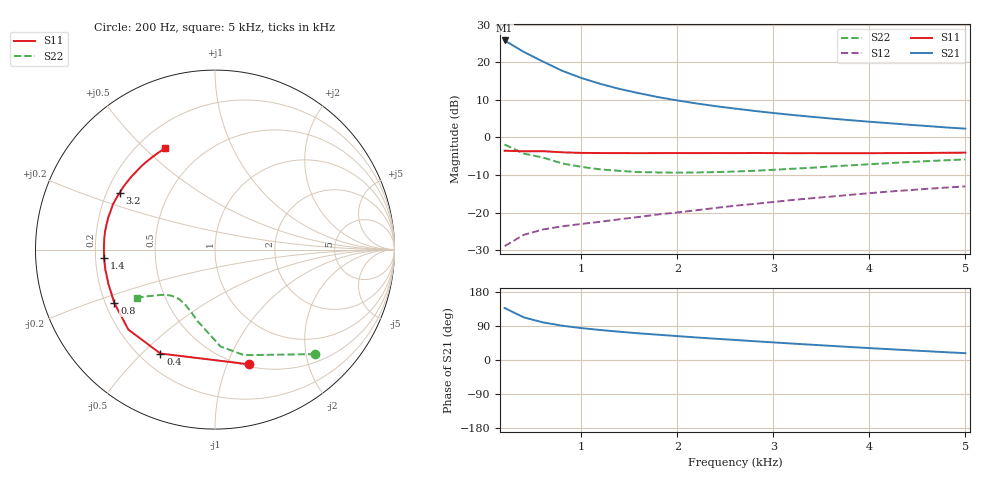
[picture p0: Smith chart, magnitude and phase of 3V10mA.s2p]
#  HZ  S  MA  R  50.0000
! Device:MCH4020
! Bias:VCE=3V, IC=10mA
!MHZ	S11(MAG/ANG)		S21(MAG/ANG)		S12(MAG/ANG)		S22(MAG/ANG)
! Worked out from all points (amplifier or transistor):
!   25 points, 200 Hz to 5 kHz, reference 50 ohm
!   highest |S21| = 25.8 dB at 200 Hz (marker M1)
!   |S21| within 3 dB of that: start of sweep to 396.7 Hz
!   unconditionally stable (mu >= 1): 2.483 kHz to 3.976 kHz
!   at 1 kHz: K = 0.59, MSG = 19.4 dB, |S12| = -23.0 dB
!   at 2.6 kHz: K = 1.01, MAG = 12.4 dB, |S12| = -18.1 dB
!   at 5 kHz: K = 0.94, MSG = 7.7 dB, |S12| = -13.0 dB
!   S11 on the Smith chart (normalised r, x): 200 Hz: 0.52, -1.20; 400 Hz: 0.28, -0.57; 800 Hz: 0.24, -0.24; 1.4 kHz: 0.23, -0.04; 3.2 kHz: 0.25, +0.26; 5 kHz: 0.31, +0.58
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200  0.667 -73.4  19.42 137.2  0.036 59.5  0.807 -46.2
400  0.654 -117.7  13.67 112.4  0.051 46.8  0.61 -74.6
600  0.657 -137.3  10.17 99.3  0.06 43.7  0.541 -86.7
800  0.635 -152.0  7.684 90.5  0.066 43.4  0.452 -96.5
1000  0.624 -162.0  6.158 84.2  0.071 44.2  0.407 -104.3
1200  0.621 -169.6  5.138 79.1  0.076 45.7  0.376 -110.1
1400  0.62 -175.7  4.4 74.5  0.082 47.0  0.36 -114.7
1600  0.619 178.9  3.867 70.4  0.088 48.7  0.347 -119.0
1800  0.62 174.4  3.431 66.7  0.095 49.8  0.343 -122.2
2000  0.621 170.6  3.103 63.0  0.101 50.9  0.341 -125.5
2200  0.62 166.6  2.828 59.5  0.108 51.7  0.343 -128.1
2400  0.621 163.0  2.602 56.1  0.116 52.3  0.347 -130.7
2600  0.62 159.4  2.419 52.9  0.124 52.6  0.353 -133.3
2800  0.622 156.1  2.253 49.6  0.131 52.8  0.361 -135.1
3000  0.62 152.7  2.112 46.5  0.139 52.8  0.372 -137.1
3200  0.618 149.2  1.99 43.3  0.148 52.6  0.384 -138.9
3400  0.619 145.6  1.881 40.3  0.156 52.3  0.396 -140.4
3800  0.618 138.5  1.696 34.3  0.173 51.2  0.426 -143.0
4200  0.62 130.9  1.549 28.6  0.191 49.6  0.456 -145.3
4600  0.623 123.4  1.419 23.2  0.208 47.7  0.485 -147.0
4800  0.626 119.8  1.359 20.5  0.216 46.7  0.498 -147.7
5000  0.629 116.2  1.309 18.0  0.224 45.6  0.511 -148.5
